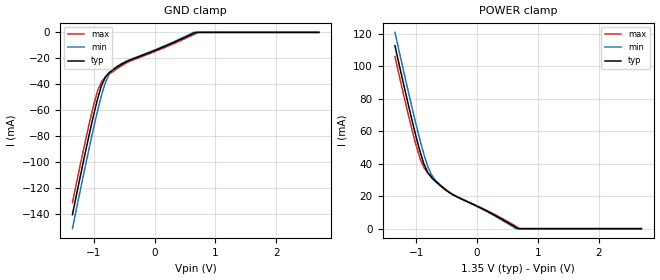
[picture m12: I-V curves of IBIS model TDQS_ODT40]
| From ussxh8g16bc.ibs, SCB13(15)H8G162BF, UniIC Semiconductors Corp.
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| MODEL TDQS_ODT40 (TDQS Terminator Model with 40ohm ODT, 800-2133Mbps)
[Model]   TDQS_ODT40
Model_type   Terminator
|   typ   min   max
|C_comp   0.965pF   0.916pF   1.023pF
C_comp_power_clamp   0.4825pF   0.4580pF   0.5115pF
C_comp_gnd_clamp   0.4825pF   0.4580pF   0.5115pF
| Note: C_comp changes when the ODT circuit is enabled.
[Voltage Range]   1.3500V   1.2830V   1.4250V
| Junction Temperature (Ambient temp is 40C typ, 85C min, 0C max)
[Temperature Range]   45.0   90.0   0.0
[GND Clamp]
|   Voltage   I(typ)   I(min)   I(max)
-1.35V    -140.6mA   -151.4mA   -131.4mA
-1.075V   -78.79mA   -89.12mA   -70.46mA
-1.005V   -64.28mA   -74.23mA   -56.57mA
-935mV    -51mA      -60.09mA   -44.75mA
-875mV    -41.28mA   -49.01mA   -38.43mA
-800mV    -33.8mA    -37.59mA   -34.26mA
-745mV    -30.93mA   -32.17mA   -32.27mA
-640mV    -27.38mA   -26.98mA   -28.74mA
-400mV    -21.26mA   -20.92mA   -22.09mA
640mV     -769.1uA   -43.14uA   -1.721mA
720mV     0A         0A         0A
2.7V      0A         0A         0A
[POWER Clamp]
|   Voltage   I(typ)   I(min)   I(max)
-1.35V    112.5mA    120.7mA    105.9mA
-1.075V   67.44mA    75.32mA    61.57mA
-935mV    47.05mA    54.01mA    42.78mA
-875mV    39.82mA    45.82mA    37.75mA
-810mV    34.41mA    38.26mA    34.36mA
-750mV    31.45mA    33.22mA    32.04mA
-690mV    29.22mA    29.94mA    29.9mA
-550mV    24.74mA    24.87mA    25.23mA
-340mV    19.7mA     19.9mA     19.86mA
640mV     765.8uA    22.39uA    1.435mA
705mV     0A         0A         0A
2.7V      0A         0A         0A
